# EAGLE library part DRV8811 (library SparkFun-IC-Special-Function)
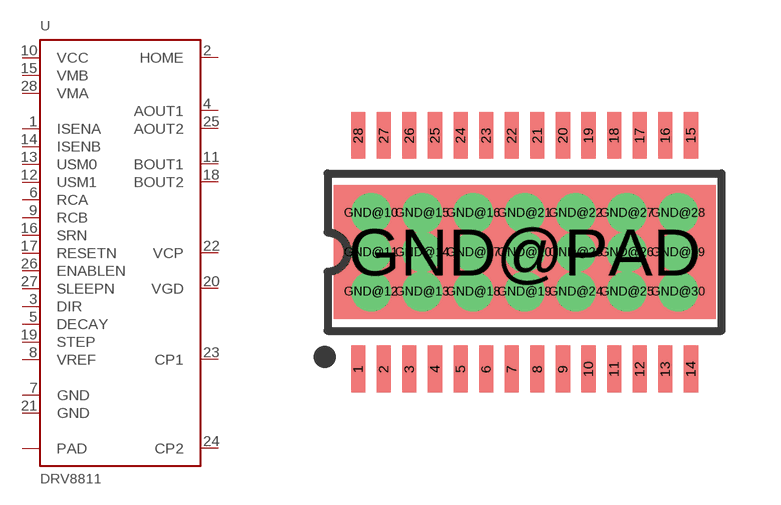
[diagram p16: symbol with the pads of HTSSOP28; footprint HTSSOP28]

Designator prefix U

## DRV8811 (PROD_ID: IC-12375)  [HTSSOP28]
1  ISENA
2  HOME
3  DIR
4  AOUT1
5  DECAY
6  RCA
7  GND
8  VREF
9  RCB
10  VCC
11  BOUT1
12  USM1
13  USM0
14  ISENB
15  VMB
16  SRN
17  RESETN
18  BOUT2
19  STEP
20  VGD
21  GND
22  VCP
23  CP1
24  CP2
25  AOUT2
26  ENABLEN
27  SLEEPN
28  VMA
GND@10  PAD
GND@11  PAD
GND@12  PAD
GND@13  PAD
GND@14  PAD
GND@15  PAD
GND@16  PAD
GND@17  PAD
GND@18  PAD
GND@19  PAD
GND@20  PAD
GND@21  PAD
GND@22  PAD
GND@23  PAD
GND@24  PAD
GND@25  PAD
GND@26  PAD
GND@27  PAD
GND@28  PAD
GND@29  PAD
GND@30  PAD
GND@PAD  PAD

## Footprint HTSSOP28 (pad centres in mm)
smd 0.36 x 1.19: 1 -4.225,-2.97; 2 -3.575,-2.97; 3 -2.925,-2.97; 4 -2.275,-2.97; 5 -1.625,-2.97; 6 -0.975,-2.97; 7 -0.325,-2.97; 8 0.325,-2.97; 9 0.975,-2.97; 10 1.625,-2.97; 11 2.275,-2.97; 12 2.925,-2.97; 13 3.575,-2.97; 14 4.225,-2.97; 15 4.225,2.97; 16 3.575,2.97; 17 2.925,2.97; 18 2.275,2.97; 19 1.625,2.97; 20 0.975,2.97; 21 0.325,2.97; 22 -0.325,2.97; 23 -0.975,2.97; 24 -1.625,2.97; 25 -2.275,2.97; 26 -2.925,2.97; 27 -3.575,2.97; 28 -4.225,2.97
drill 0.508: GND@10 -3.9,1; GND@11 -3.9,0; GND@12 -3.9,-1; GND@13 -2.6,-1; GND@14 -2.6,0; GND@15 -2.6,1; GND@16 -1.3,1; GND@17 -1.3,0; GND@18 -1.3,-1; GND@19 0,-1; GND@20 0,0; GND@21 0,1; GND@22 1.3,1; GND@23 1.3,0; GND@24 1.3,-1; GND@25 2.6,-1; GND@26 2.6,0; GND@27 2.6,1; GND@28 3.9,1; GND@29 3.9,0; GND@30 3.9,-1
smd 9.7 x 3.4: GND@PAD 0,0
